(* Logix 5000 AddOnInstructionDefinition export FB_DRVI_EIP_1_0; software revision 37.00 *)

TYPE UDT_DRVI_DataInput :
STRUCT
   inStatusWord : INT;
   inOperatingModeState : INT;
   diDiagnosticWarning : INT;
   diDiagnostiError : INT;
   diActualSpeed : DINT;
   diActualPosition : DINT;
   inActualTorqueCurrent : INT;
   inGPIO_DigInputStatus : INT;
END_STRUCT
END_TYPE

TYPE UDT_DRVI_DataOutput :
STRUCT
   inControlWord : INT;
   inOperatingMode : INT;
   inGPIO_DigOutput : INT;
   diTargetPosition : DINT;
   diTargetSpeed : DINT;
   inTargetAccel : INT;
   inTargetDecel : INT;
   inTargetTorque : INT;
END_STRUCT
END_TYPE

ADD_ON_INSTRUCTION FB_DRVI_EIP_1_0   (* revision 1.0, vendor Camozzi spa *)
// Camozzi Servodrive DRVI EIP
// Revision note:
// Version.Release 33.0 July 2025
// Help:
// ////////////////////////////////////////////////////////////
// //   Copyright (c)  Camozzi spa (Italy)
// //------------------------------------------------------------
// //   FB AOI: FB_DRVI
// //   Author: S.M./D.F.
// //   Created: 26/07/2025
// //   Version.Release: 33.0 (July 2025)
// //------------------------------------------------------------
// //   Function Block Description:
// //
// //   The FB_DRVI Add On Instruction (AOI) is a function block
// //   to manage DRVI servodrive
// //
// //
// //------------------------------------------------------------
// //   Version History: None
// //   v33.0 - 1st version
// //
// ////////////////////////////////////////////////////////////
VAR_INPUT
   I_boServoOffOn : BOOL; {visible}
   I_boClearError : BOOL; {visible}
   I_boStartMove : BOOL; {visible}   // Starts move command, speed, pos, jog, torque, homing
   I_boStopMove : BOOL; {visible}   // Stops any motion in progress
   I_boQuickStopMove : BOOL; {visible}   // Stops any motion in progress
   I_boJogLeft : BOOL; {visible}
   I_boJogRight : BOOL; {visible}
   I_boSwLim : BOOL; {visible}
   I_boTorqLim : BOOL; {visible}
   I_inOperatingMode : INT; {visible}   // Operating mode setting: 0= none, 1= Speed, 2= Rel pos, 3= Abs pos, 4= Torque, 5 to 13= Homing 0 to 8, 14= Jog
   I_reTargetSpeed_RPM : REAL; {visible}
   I_reTargetPosition_deg : REAL; {visible}
   I_inTargetAccel_units_sec : INT; {visible}
   I_inTargetDecel_units_sec : INT; {visible}
   I_siTorque_ma : INT; {visible}
   I_bo_GPIO_Out_0 : BOOL; {visible}
END_VAR
VAR_IN_OUT
   _DRVI_InstanceName : MODULE; {required}   // Map to DRVI module
   _DRVI_I_Data : SINT[20]; {required}   // Map to DRVI module input data
   _DRVI_O_Data : SINT[20]; {required}   // Map to DRVI module output data
END_VAR
VAR_OUTPUT
   Q_boCommUp : BOOL; {access Read Only, visible}   // Module Communication State is Running
   Q_boCommInhibited : BOOL; {access Read Only}   // Module Communication State is Inhibited
   Q_boCommDown : BOOL; {access Read Only}   // Module Communication State is Error
   Q_boStartMoveCmdActive : BOOL; {access Read Only, visible}
   Q_boDriveStatus_ServoOn : BOOL; {access Read Only, visible}
   Q_boDriveStatus_Busy : BOOL; {access Read Only, visible}
   Q_boDriveStatus_TargetReached : BOOL; {access Read Only, visible}
   Q_boDriveStatus_Error : BOOL; {access Read Only, visible}
   Q_boDriveStatus_JogRight : BOOL; {access Read Only, visible}
   Q_boDriveStatus_JogLeft : BOOL; {access Read Only, visible}
   Q_boDriveStatus_HomingDone : BOOL; {access Read Only, visible}
   Q_boDriveStatus_UvixManModeActive : BOOL; {access Read Only, visible}
   Q_boDriveStatus_SoftwareLimit : BOOL; {access Read Only, visible}
   Q_boDriveStatus_TorqueLimit : BOOL; {access Read Only, visible}
   Q_inActOperatingMode : INT; {visible}
END_VAR
VAR_IN_OUT
   Q_stActOperatingMode : STRING; {required}
END_VAR
VAR_OUTPUT
   Q_reActualPosition_deg : REAL; {access Read Only, visible}
   Q_reActualSpeed_RPM : REAL; {access Read Only, visible}
   Q_inActualTorque_mA : INT; {access Read Only, visible}
   Q_inWarning : INT; {access Read Only, visible}
   Q_inError : INT; {access Read Only, visible}
   Q_boGPIO_IN_0 : BOOL; {access Read Only, visible}
   Q_boGPIO_IN_1 : BOOL; {access Read Only, visible}
   Q_boGPIO_ExtProxy : BOOL; {access Read Only, visible}
   Q_boGPIO_HomeProxy : BOOL; {access Read Only, visible}
END_VAR
VAR_IN_OUT
   Q_stWarning : STRING; {required}
   Q_stError : STRING; {required}
END_VAR
VAR
   diModuleCommStatus : DINT; {access None}
   udtDRVI_DataIn : UDT_DRVI_DataInput; {access None}
   aysiCopyDataIn : SINT[20]; {access None}
   diIndex : DINT; {access None}
   stDummyString : STRING; {access None}
   udtDRVI_DataOut : UDT_DRVI_DataOutput; {access None}
END_VAR

ROUTINE Logic   (* structured text *)
   ////////////////////////////////////////////////////////////
   //   Copyright (c)  Camozzi spa (Italy)
   //------------------------------------------------------------
   //   FB AOI: FB_DRVI
   //   Author: S.M./D.F.
   //   Created: 08/05/2026
   //   Version.Release: 1.0 (May 2026)
   //------------------------------------------------------------
   //   Function Block Description:
   //
   //   The FB_DRVI Add On Instruction (AOI) is a function block
   //   to manage DRVI servodrive
   //
   //
   //------------------------------------------------------------
   //   Version History: None
   //   v1.0 - 1st version
   //
   ////////////////////////////////////////////////////////////
   
   
   // === Communication status ===
   GSV(Module,_DRVI_InstanceName,EntryStatus,diModuleCommStatus);
   
   IF (diModuleCommStatus = 16384) THEN
   	Q_boCommUp := 1;
   	Q_boCommInhibited := 0;
   	Q_boCommDown := 0;
   ELSIF (diModuleCommStatus = 24576) THEN
   	Q_boCommUp := 0;
   	Q_boCommInhibited := 1;
   	Q_boCommDown := 0;
   ELSE
   	Q_boCommUp := 0;
   	Q_boCommInhibited := 0;
   	Q_boCommDown := 1;
   END_IF;
   
   IF Q_boCommUp THEN
   	CPS(_DRVI_I_Data[0],udtDRVI_DataIn,1);
   ELSE
   	FOR diIndex := 0 TO 19 DO
   		aysiCopyDataIn[diIndex] := 0;
   		CPS(aysiCopyDataIn[0],udtDRVI_DataIn,28);
   	END_FOR;
   END_IF;
   
   
   // === Actual operating mode decoding ===
   Q_inActOperatingMode := udtDRVI_DataIn.inOperatingModeState;
   COP(stDummyString,Q_stActOperatingMode,1);
   CASE udtDRVI_DataIn.inOperatingModeState OF
   	1:
   		Q_stActOperatingMode := 'speed';
   
   	2:
   		Q_stActOperatingMode := 'rel_pos';
   
   	3:
   		Q_stActOperatingMode := 'abs_pos';
   
   	4:
   		Q_stActOperatingMode := 'torque';
   
   	5:
   		Q_stActOperatingMode := 'homing_stand';
   
   	6:
   		Q_stActOperatingMode := 'homing_proxy_left';
   
   	7:
   		Q_stActOperatingMode := 'homing_proxy_right';
   
   	8:
   		Q_stActOperatingMode := 'homing_proxy_zero_left';
   
   	9:
   		Q_stActOperatingMode := 'homing_proxy_zero_right';
   
   	10:
   		Q_stActOperatingMode := 'homing_torque_left';
   
   	11:
   		Q_stActOperatingMode := 'homing_torque_right';
   
   	12:
   		Q_stActOperatingMode := 'homing_torque_zero_left';
   
   	13:
   		Q_stActOperatingMode := 'homing_torque_zero_right';
   
   	14:
   		Q_stActOperatingMode := 'jog';
   
   ELSE
   	Q_stActOperatingMode := 'none';
   
   END_CASE;
   
   
   // === Drive status and monitoring data ===
   Q_boDriveStatus_ServoOn := udtDRVI_DataIn.inStatusWord.0;
   Q_boDriveStatus_Busy := udtDRVI_DataIn.inStatusWord.1;
   Q_boDriveStatus_TargetReached := udtDRVI_DataIn.inStatusWord.2;
   Q_boDriveStatus_Error := udtDRVI_DataIn.inStatusWord.3;
   Q_boDriveStatus_HomingDone := udtDRVI_DataIn.inStatusWord.4;
   Q_boDriveStatus_UvixManModeActive := NOT udtDRVI_DataIn.inStatusWord.5;
   Q_boDriveStatus_SoftwareLimit := udtDRVI_DataIn.inStatusWord.6;
   Q_boDriveStatus_TorqueLimit := udtDRVI_DataIn.inStatusWord.7;
   Q_boDriveStatus_JogLeft := udtDRVI_DataIn.inStatusWord.8;
   Q_boDriveStatus_JogRight := udtDRVI_DataIn.inStatusWord.9;
   Q_reActualPosition_deg := udtDRVI_DataIn.diActualPosition / 100;
   Q_reActualSpeed_RPM := udtDRVI_DataIn.diActualSpeed / 100;
   Q_inActualTorque_mA := udtDRVI_DataIn.inActualTorqueCurrent;
   
   
   // === Update  GIIO IN
   if ( udtDRVI_DataIn.inGPIO_DigInputStatus AND 1 ) > 0 then
   	Q_boGPIO_IN_0 := 1;
   else
   	Q_boGPIO_IN_0 := 0;
   end_if;
   
   if ( udtDRVI_DataIn.inGPIO_DigInputStatus AND 2 ) > 0 then
   	Q_boGPIO_IN_1 := 1;
   else
   	Q_boGPIO_IN_1 := 0;
   end_if;
   
   if ( udtDRVI_DataIn.inGPIO_DigInputStatus AND 4 ) > 0 then
   	Q_boGPIO_ExtProxy := 1;
   else
   	Q_boGPIO_ExtProxy := 0;
   end_if;
   
   if ( udtDRVI_DataIn.inGPIO_DigInputStatus AND 8 ) > 0 then
   	Q_boGPIO_HomeProxy := 1;
   else
   	Q_boGPIO_HomeProxy := 0;
   end_if;
   
   
   // === Warning and error status ===
   Q_inError := udtDRVI_DataIn.diDiagnostiError;
   Q_inWarning := udtDRVI_DataIn.diDiagnosticWarning;
   
   // decode error
   COP(stDummyString,Q_stError,1);
   IF ( Q_inError AND 1) > 0 then
   	Q_stError := 'VDC UVLO';
   end_if;
   
   IF ( Q_inError AND 2) > 0 then
   	Q_stError := 'VDC OVLO';
   end_if;
   
   IF ( Q_inError AND 4) > 0 then
   	Q_stError := 'VL UVLO';
   end_if;
   
   IF ( Q_inError AND 8) > 0 then
   	Q_stError := 'VL OVLO';
   end_if;
   
   IF ( Q_inError AND 16) > 0 then
   	Q_stError := 'Motor Overtemperature';
   end_if;
   
   IF ( Q_inError AND 32) > 0 then
   	Q_stError := 'Drive Overtemperature';
   end_if;
   
   IF ( Q_inError AND 64) > 0 then
   	Q_stError := 'Current sensor';
   end_if;
   
   IF ( Q_inError AND 128) > 0 then
   	Q_stError := 'Control loop';
   end_if;
   
   IF ( Q_inError AND 256) > 0 then
   	Q_stError := 'Encoder fail';
   end_if;
   
   IF ( Q_inError AND 512) > 0 then
   	Q_stError := 'Memory fail';
   end_if;
   
   IF ( Q_inError AND 1024) > 0 then
   	Q_stError := 'I2T';
   end_if;
   
   IF ( Q_inError AND 2048) > 0 then
   	Q_stError := 'STO';
   end_if;
   
   IF ( Q_inError AND 4096) > 0 then
   	Q_stError := 'Homing execution';
   end_if;
   
   IF ( Q_inError AND 8192) > 0 then
   	Q_stError := 'Software limit';
   end_if;
   
   
   // decode warning
   COP(stDummyString,Q_stWarning,1);
   IF ( Q_inWarning AND 1) > 0 then
   	Q_stWarning := 'VDC UVLO';
   end_if;
   
   IF ( Q_inWarning AND 2) > 0 then
   	Q_stWarning := 'VDC OVLO';
   end_if;
   
   IF ( Q_inWarning AND 4) > 0 then
   	Q_stWarning := 'VL UVLO';
   end_if;
   
   IF ( Q_inWarning AND 8) > 0 then
   	Q_stWarning := 'VL OVLO';
   end_if;
   
   IF ( Q_inWarning AND 16) > 0 then
   	Q_stWarning := 'Motor Overtemperature';
   end_if;
   
   IF ( Q_inWarning AND 32) > 0 then
   	Q_stWarning := 'Drive Overtemperature';
   end_if;
   
   IF ( Q_inWarning AND 64) > 0 then
   	Q_stWarning := 'Calibration missed';
   end_if;
   
   IF ( Q_inWarning AND 256) > 0 then
   	Q_stWarning := 'Homing not done';
   end_if;
   
   IF ( Q_inWarning AND 512) > 0 then
   	Q_stWarning := 'Speed target not reached';
   end_if;
   
   IF ( Q_inWarning AND 1024) > 0 then
   	Q_stWarning := 'Position target not reached';
   end_if;
   
   
   IF ( Q_inWarning AND 2048) > 0 then
   	Q_stWarning := 'Command refused';
   end_if;
   
   
   // === Control Commands ===
   udtDRVI_DataOut.inControlWord := 0;
   
   IF I_boClearError THEN
       udtDRVI_DataOut.inControlWord.4 := 1;
   ELSE
       udtDRVI_DataOut.inControlWord.4 := 0;
   END_IF;
   
   
   IF I_boServoOffOn THEN
       udtDRVI_DataOut.inControlWord.0 := 1;
   ELSE
       udtDRVI_DataOut.inControlWord.0 := 0;
   END_IF;
   
   
   IF I_boStartMove AND Q_boCommUp AND Q_boDriveStatus_ServoOn AND (NOT Q_boDriveStatus_UvixManModeActive)
   	AND (udtDRVI_DataIn.inOperatingModeState > 0) AND (Q_inError = 0 ) AND (NOT I_boStopMove) AND (NOT I_boQuickStopMove) THEN
       udtDRVI_DataOut.inControlWord.1 := 1;
       Q_boStartMoveCmdActive := 1;
   ELSE
       udtDRVI_DataOut.inControlWord.1 := 0;
       Q_boStartMoveCmdActive := 0;
   END_IF;
   
   
   IF I_boStopMove THEN
       udtDRVI_DataOut.inControlWord.2 := 1;
   ELSE
       udtDRVI_DataOut.inControlWord.2 := 0;
   END_IF;
   
   
   IF I_boQuickStopMove THEN
       udtDRVI_DataOut.inControlWord.3 := 1;
   ELSE
       udtDRVI_DataOut.inControlWord.3 := 0;
   END_IF;
   
   
   IF I_boSwLim THEN
       udtDRVI_DataOut.inControlWord.6 := 1;
   ELSE
       udtDRVI_DataOut.inControlWord.6 := 0;
   END_IF;
   
   
   IF I_boTorqLim THEN
       udtDRVI_DataOut.inControlWord.7 := 1;
   ELSE
       udtDRVI_DataOut.inControlWord.7 := 0;
   END_IF;
   
   
   // === Jog ===
   IF (udtDRVI_DataIn.inOperatingModeState >= 2) AND Q_boDriveStatus_ServoOn THEN
       IF I_boJogLeft AND (NOT I_boJogRight) THEN
           udtDRVI_DataOut.inControlWord.8 := 1;
           udtDRVI_DataOut.inControlWord.9 := 0;
       ELSIF (NOT I_boJogLeft) AND I_boJogRight THEN
           udtDRVI_DataOut.inControlWord.8 := 0;
           udtDRVI_DataOut.inControlWord.9 := 1;
       ELSE
           udtDRVI_DataOut.inControlWord.8 := 0;
           udtDRVI_DataOut.inControlWord.9 := 0;
       END_IF;
   ELSE
       udtDRVI_DataOut.inControlWord.8 := 0;
       udtDRVI_DataOut.inControlWord.9 := 0;
   END_IF;
   
   
   // === Output setting data ===
   udtDRVI_DataOut.inOperatingMode := I_inOperatingMode;
   udtDRVI_DataOut.inTargetAccel := I_inTargetAccel_units_sec;
   udtDRVI_DataOut.inTargetDecel := I_inTargetDecel_units_sec;
   udtDRVI_DataOut.diTargetSpeed := I_reTargetSpeed_RPM * 100;
   udtDRVI_DataOut.diTargetPosition := I_reTargetPosition_deg * 100;
   udtDRVI_DataOut.inTargetTorque := I_siTorque_ma;
   if I_bo_GPIO_Out_0 then
   	udtDRVI_DataOut.inGPIO_DigOutput := 1;
   else
   	udtDRVI_DataOut.inGPIO_DigOutput := 0;
   end_if;
   
   
   IF Q_boCommUp THEN
   	// === Output data mapping ===
   	CPS(udtDRVI_DataOut.inControlWord,_DRVI_O_Data[0],2);
   	CPS(udtDRVI_DataOut.inOperatingMode,_DRVI_O_Data[2],2);
   	CPS(udtDRVI_DataOut.inGPIO_DigOutput,_DRVI_O_Data[4],2);
   	CPS(udtDRVI_DataOut.diTargetPosition,_DRVI_O_Data[6],4);
   	CPS(udtDRVI_DataOut.diTargetSpeed,_DRVI_O_Data[10],4);
   	CPS(udtDRVI_DataOut.inTargetAccel,_DRVI_O_Data[14],2);
   	CPS(udtDRVI_DataOut.inTargetDecel,_DRVI_O_Data[16],2);
   	CPS(udtDRVI_DataOut.inTargetTorque,_DRVI_O_Data[18],2);
   end_if;
   
   
   // End Prog
END_ROUTINE
END_ADD_ON_INSTRUCTION
